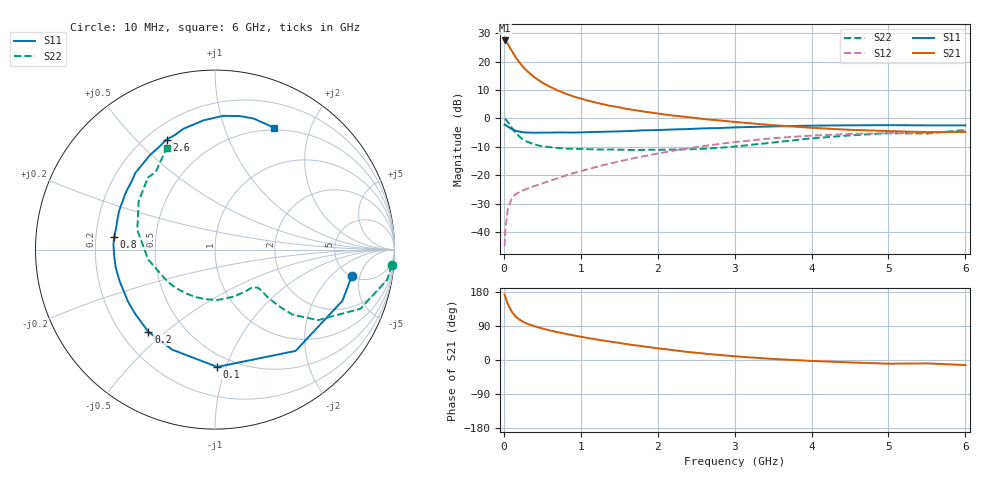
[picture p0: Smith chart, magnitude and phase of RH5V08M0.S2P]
! SIEMENS Small Signal Semiconductors
! BFR106
! Si NPN RF Bipolar Junction Transistor in SOT23
! VCE = 5 V  IC = 8 mA
! Common Emitter S-Parameters:  August  1996
# GHz  S  MA  R  50
!  f  S11  S21  S12  S22
! GHz  MAG  ANG  MAG  ANG  MAG  ANG  MAG  ANG
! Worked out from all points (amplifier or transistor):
!   36 points, 10 MHz to 6 GHz, reference 50 ohm
!   highest |S21| = 27.5 dB at 10 MHz (marker M1)
!   |S21| within 3 dB of that: start of sweep to 89.47 MHz
!   unconditionally stable (mu >= 1): 534.9 MHz to 1.969 GHz; 5.16 GHz to end of sweep
!   at 250 MHz: K = 0.64, MSG = 21.8 dB, |S12| = -25.4 dB
!   at 1.4 GHz: K = 1.11, MAG = 8.1 dB, |S12| = -15.8 dB
!   at 6 GHz: K = 1.01, MAG = -0.8 dB, |S12| = -4.5 dB
!   S11 on the Smith chart (normalised r, x): 10 MHz: 5.09, -3.76; 100 MHz: 0.41, -0.93; 200 MHz: 0.31, -0.44; 800 MHz: 0.28, +0.06; 2.6 GHz: 0.28, +0.62; 6 GHz: 0.47, +1.49
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0.01  0.7761 -10.9  23.72 172.5  0.0056 86.9  0.9876 -4.9
0.02  0.7651 -21.9  23.32 166.5  0.0107 81.6  0.9742 -9.9
0.05  0.7213 -51.5  20.58 148.6  0.0246 66.1  0.8753 -22.1
0.1  0.6537 -88.9  15.9 128.6  0.0384 53.2  0.6956 -34.4
0.15  0.6065 -113.2  12.22 115.1  0.0458 46.5  0.5633 -40.0
0.2  0.5896 -129.0  9.838 107.1  0.05 44.9  0.4831 -41.4
0.25  0.571 -141.0  8.11 100.6  0.054 44.6  0.4246 -41.9
0.3  0.5649 -149.0  6.889 96.2  0.0574 45.7  0.3907 -42.1
0.4  0.5598 -161.7  5.296 89.1  0.0644 48.4  0.3464 -41.4
0.5  0.5623 -170.1  4.272 83.1  0.0716 51.5  0.3234 -41.5
0.6  0.5628 -177.1  3.61 77.9  0.0797 54.2  0.3111 -42.6
0.8  0.5657 172.7  2.75 69.2  0.0983 58.1  0.294 -46.5
0.9  0.5639 167.7  2.458 65.2  0.1081 59.7  0.2914 -48.5
1.1  0.5745 159.1  2.056 57.7  0.1283 61.6  0.287 -54.9
1.3  0.5814 151.7  1.767 51.2  0.151 62.3  0.2821 -61.5
1.6  0.597 142.1  1.47 41.8  0.1873 62.1  0.2793 -73.4
2.2  0.6393 124.6  1.124 26.0  0.2694 57.5  0.282 -101.3
2.6  0.6694 113.8  0.977 17.1  0.3262 52.3  0.2924 -123.2
3.5  0.7234 94.9  0.761 2.7  0.4489 37.4  0.3764 -171.5
4.5  0.7566 79.5  0.63 -6.4  0.5313 19.1  0.5027 147.9
5.5  0.755 67.9  0.574 -8.9  0.5636 7.0  0.5436 127.5
6  0.7538 64.1  0.58 -13.4  0.5946 -1.0  0.6268 115.5
